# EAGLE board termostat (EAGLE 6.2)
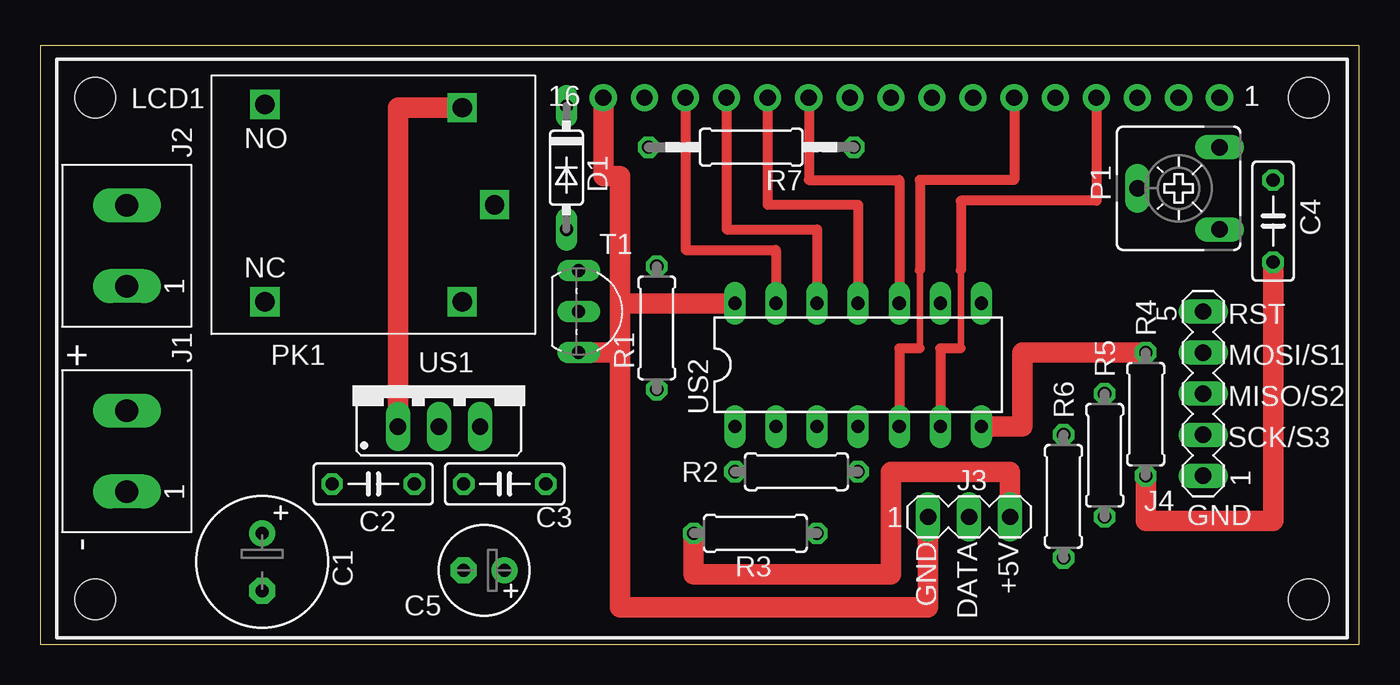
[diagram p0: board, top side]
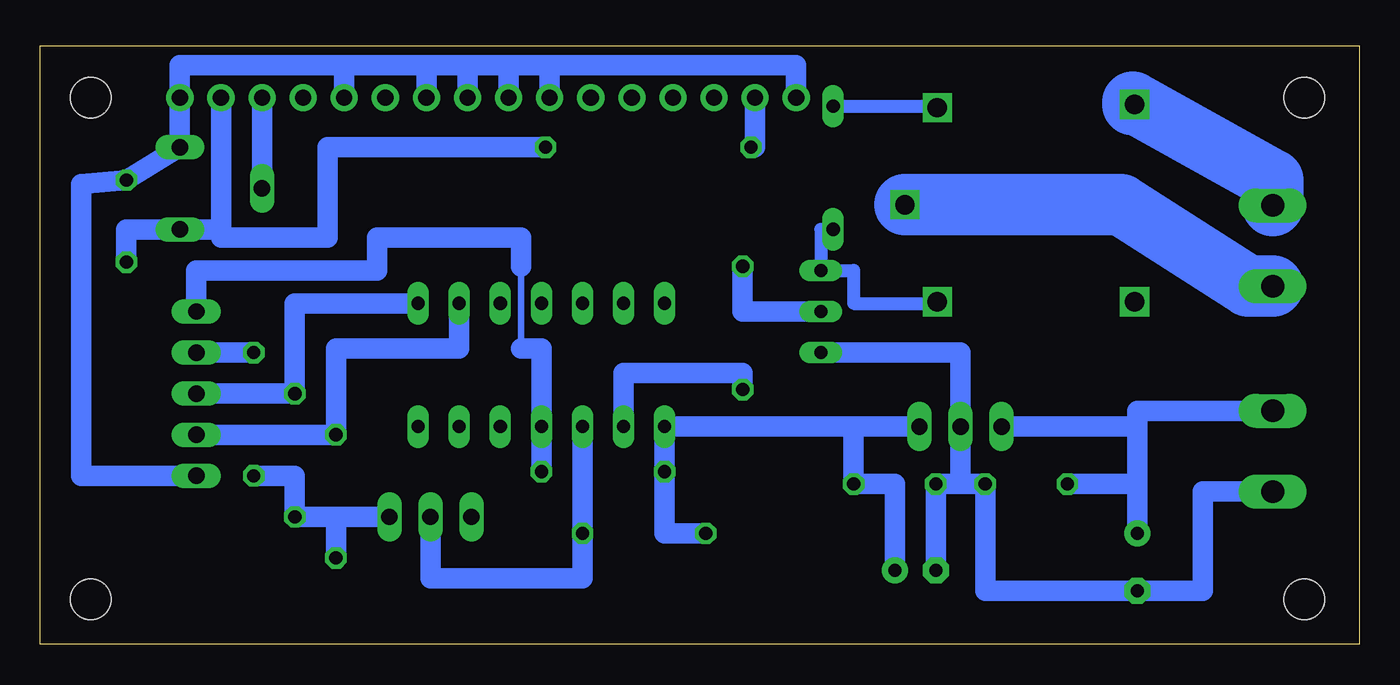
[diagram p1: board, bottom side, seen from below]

Size 81.51 x 37.01 mm. Coordinates in mm from the lower left corner, seen from the top.
Outline: 0,0 81.51,0 81.51,37.01 0,37.01 0,0
Copper layers (1*16): Top 0.035mm / dielectric 1.5mm / Bottom 0.035mm
Design rules: minimum track width 10mil, minimum drill 24mil, track to track 8mil, track to pad 8mil, pad to pad 8mil, via to via 8mil, smd to smd 8mil, copper to edge 40mil, drill to drill 8mil, minimum pad ring 10mil, minimum via ring 8mil, stop-mask expansion 4mil, vias tented up to drill 0mil, thermal gap 10mil

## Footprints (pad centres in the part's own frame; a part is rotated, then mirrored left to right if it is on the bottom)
E3,5-8 = drill 0.813 pad 1.6: + -1.778,0 | drill 0.813 pad 1.6 octagon: - 1.778,0
C050-025X075 = drill 0.813 octagon: 1 -2.54,0; 2 2.54,0
E2,5-6 = drill 0.813 pad 1.6: + -1.27,0 | drill 0.813 pad 1.6 octagon: - 1.27,0
DO35-7 = drill 0.813 long: A 3.81,0; C -3.81,0
2PIN-5MM = drill 1.4 long: P$1 -2.5,0; P$2 2.5,0
MA03-1 = drill 1.016 long: 1 -2.54,0; 2 0,0; 3 2.54,0
MA05-1 = drill 1.016 long: 1 -5.08,0; 2 -2.54,0; 3 0,0; 4 2.54,0; 5 5.08,0
LCD_HD44780_2X16_POD-SCIEZKAMI = drill 1 pad 1.676: 1 32,15.5; 2 29.46,15.5; 3 26.92,15.5; 4 24.38,15.5; 5 21.84,15.5; 6 19.3,15.5; 7 16.76,15.5; 8 14.22,15.5; 9 11.68,15.5; 10 9.14,15.5; 11 6.6,15.5; 12 4.06,15.5; 13 1.52,15.5; 14 -1.02,15.5; 15 -3.56,15.5; 16 -6.1,15.5 | hole 2.5: -37.5,-15.5; 37.5,-15.5; -37.5,15.5; 37.5,15.5
CA6V = drill 1.016 long: A -2.54,-2.54; E 2.54,-2.54; S 0,2.54
PK_POJED_JQC-3FG = drill 1.2 square: 1 5.5,6; 2 5.5,-6; C 7.5,0; NC -6.7,-6; NO -6.7,6.2
0207/7 = drill 0.813 octagon: 1 -3.81,0; 2 3.81,0
0207/12 = drill 0.813 octagon: 1 -6.35,0; 2 6.35,0
TO92-EBC = drill 0.813 long: B 0,-1.27; C -2.54,-1.27; E 2.54,-1.27
78XXS = drill 1.016 long: GND 0,-2.54; IN -2.54,-2.54; OUT 2.54,-2.54
DIL14 = drill 0.813 long: 1 -7.62,-3.81; 2 -5.08,-3.81; 3 -2.54,-3.81; 4 0,-3.81; 5 2.54,-3.81; 6 5.08,-3.81; 7 7.62,-3.81; 8 7.62,3.81; 9 5.08,3.81; 10 2.54,3.81; 11 0,3.81; 12 -2.54,3.81; 13 -5.08,3.81; 14 -7.62,3.81

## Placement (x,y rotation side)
C1  220u/35V  [E3,5-8]  13.72,5.08 270 top
C2  100n  [C050-025X075]  20.57,9.91 0 top
C3  100n  [C050-025X075]  28.7,9.91 180 top
C4  100n  [C050-025X075]  76.2,26.16 90 top
C5  100u/16V  [E2,5-6]  27.43,4.57 180 top
D1  1N4148  [DO35-7]  32.51,29.46 270 top
J1  ARK2-5MM  [2PIN-5MM]  5.33,11.94 90 top
J2  ARK2-5MM  [2PIN-5MM]  5.33,24.64 90 top
J3  [MA03-1]  57.4,7.87 0 top
J4  [MA05-1]  71.88,15.49 90 top
LCD1  1x16  [LCD_HD44780_2X16_POD-SCIEZKAMI]  40.89,18.29 0 top
P1  10k  [CA6V]  70.36,28.19 90 top
PK1  JQC-3FG  [PK_POJED_JQC-3FG]  20.57,27.18 0 top
R1  3,3k  [0207/7]  38.1,19.56 90 top
R2  3,3k  [0207/7]  46.74,10.67 180 top
R3  3,3k  [0207/7]  44.2,6.86 180 top
R4  3,3k  [0207/7]  68.33,14.22 90 top
R5  3,3k  [0207/7]  65.79,11.68 90 top
R6  3,3k  [0207/7]  63.25,9.14 90 top
R7  47  [0207/12]  43.94,30.73 180 top
T1  BC546  [TO92-EBC]  34.54,20.57 270 top
US1  7805  [78XXS]  24.64,16 0 top
US2  ATTINY24/44/84-PU  [DIL14]  50.55,17.27 0 top

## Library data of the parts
C1-C5 R1-R7 = rcl
D1 = diode
J1 J2 = zlacza_futrzak
J3 J4 = con-lstb; OC_FARNELL: unknown; OC_NEWARK: unknown
LCD1 PK1 = inne_futrzak
P1 = pot
T1 = transistor-npn
US1 = v-reg
US2 = scalaki_futrzak

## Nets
+5V: C3.1 C4.1 C5.+ J3.3 LCD1.2 P1.A R2.2 R3.2 R4.1 R5.1 R6.1 R7.1 US1.OUT US2.1
GND: C1.- C2.2 C3.2 C4.2 C5.- J1.P$1 J3.1 J4.1 LCD1.1 LCD1.5 LCD1.7 LCD1.8 LCD1.9 LCD1.10 LCD1.16 P1.E T1.E US1.GND US2.14
N$1: J4.5 R2.1 US2.4
N$31: C1.+ C2.1 D1.C J1.P$2 PK1.1 US1.IN
N$33: J2.P$2 PK1.NO
N$34: J2.P$1 PK1.C
N$35: J4.2 R6.2 US2.9
N$36: D1.A PK1.2 T1.C
N$38: J4.3 R5.2 US2.8
N$39: J3.2 R3.1 US2.3
N$40: J4.4 R4.2 US2.7
N$48: LCD1.3 P1.S
N$49: LCD1.15 R7.2
N$50: LCD1.14 US2.13
N$51: LCD1.13 US2.12
N$52: LCD1.4 US2.6
N$53: LCD1.6 US2.5
N$54: LCD1.12 US2.11
N$55: LCD1.11 US2.10
N$56: R1.2 T1.B
N$57: R1.1 US2.2

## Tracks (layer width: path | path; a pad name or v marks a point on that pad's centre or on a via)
+5V
  Top 1.27: R4.1 68.33,7.62 76.2,7.62 C4.1 | J3.3 59.94,10.67 52.58,10.67 52.58,4.32 40.39,4.32 R3.2
  Bottom 1.27: US1.OUT 31.24,13.46 | 31.24,13.46 C3.1 28.7,9.91 C5.+ | 31.24,13.46 US2.1 R2.2 42.93,6.86 R3.2 | 70.35,25.65 P1.A 76.2,25.65 C4.1 | 70.35,25.65 LCD1.2 | R4.1 65.79,10.41 R5.1 63.25,7.87 | R7.1 63.75,30.73 63.75,25.15 70.35,25.15 70.35,25.65 | J3.3 63.25,7.87 | 63.25,7.87 R6.1
GND
  Top 1.27: T1.E 35.81,18.03 | 35.81,18.03 35.81,21.08 | 35.81,21.08 35.81,28.96 34.79,28.96 LCD1.16 | US2.14 35.81,21.08 | J3.1 54.86,2.29 35.81,2.29 35.81,18.03
  Bottom 1.27: J1.P$1 9.65,9.44 9.65,3.3 C1.- 23.11,3.3 C2.2 24.64,9.91 | 24.64,9.91 C3.2 C5.- | 24.64,9.91 US1.GND 24.64,18.03 T1.E | 62.74,35.81 72.9,35.81 LCD1.1 72.89,30.99 P1.E C4.2 78.99,28.45 78.99,10.41 J4.1 | 62.74,35.81 62.73,35.81 | 62.73,35.81 LCD1.5 62.74,35.81 | 62.73,35.81 57.66,35.81 | 57.66,35.81 57.65,35.81 | 57.65,35.81 LCD1.7 57.66,35.81 | 57.65,35.81 55.12,35.81 | 55.12,35.81 55.11,35.81 | 55.11,35.81 LCD1.8 55.12,35.81 | 55.11,35.81 52.58,35.81 | 52.58,35.81 52.57,35.81 | 52.57,35.81 LCD1.9 52.58,35.81 | 52.57,35.81 50.04,35.81 | 50.04,35.81 50.03,35.81 | 50.03,35.81 LCD1.10 50.04,35.81 | 50.03,35.81 34.79,35.81 LCD1.16
N$1
  Bottom 0.406: 51.82,23.37 51.82,18.29
  Bottom 1.27: R2.1 US2.4 50.55,18.29 51.82,18.29 | J4.5 71.88,23.11 60.71,23.11 60.71,25.15 51.82,25.15 51.82,23.37
N$31
  Top 1.27: PK1.1 22.1,33.18 US1.IN
  Bottom 0.813: D1.C 26.07,33.27 PK1.1
  Bottom 1.27: J1.P$2 13.72,14.44 13.72,13.46 | 13.72,9.91 C1.+ | C2.1 13.72,9.91 | 13.72,9.91 13.72,13.46 | 13.72,13.46 US1.IN
N$33
  Bottom 3.81: PK1.NO 13.97,33.38 13.97,33.53 5.33,28.7 J2.P$2
N$34
  Bottom 3.81: J2.P$1 6.86,22.14 14.73,27.18 PK1.C
N$35
  Bottom 1.27: J4.2 R6.2 63.25,18.29 55.63,18.29 US2.9
N$36
  Bottom 0.813: D1.A 33.27,25.65 T1.C 31.24,23.11 31.24,21.08 26.16,21.08 26.16,21.34 26.07,21.34 PK1.2
N$38
  Bottom 1.27: J4.3 R5.2 65.79,21.08 US2.8
N$39
  Bottom 1.27: US2.3 R3.1 48.01,4.06 57.4,4.06 J3.2
N$40
  Top 1.27: R4.2 60.71,18.03 60.71,13.46 US2.7
  Bottom 1.27: J4.4 R4.2
N$48
  Bottom 1.27: P1.S 67.81,29.72 LCD1.3
N$49
  Bottom 1.27: R7.2 37.33,30.73 LCD1.15
N$50
  Top 0.61: LCD1.14 39.88,24.38 45.47,24.38 US2.13
N$51
  Top 0.61: LCD1.13 42.42,25.65 48.01,25.65 US2.12
N$52
  Top 0.406: 56.9,23.11 56.9,18.29
  Top 0.61: LCD1.4 65.28,27.43 56.9,27.43 56.9,23.11 | 56.9,18.29 55.63,18.29 US2.6
N$53
  Top 0.406: 54.36,23.11 54.36,18.29
  Top 0.61: LCD1.6 60.2,28.7 54.36,28.7 54.36,23.11 | 54.36,18.29 53.09,18.29 US2.5
N$54
  Top 0.61: LCD1.12 44.96,27.18 50.55,27.18 US2.11
N$55
  Top 0.61: LCD1.11 47.5,28.7 53.09,28.7 US2.10
N$56
  Bottom 1.27: T1.B 38.1,20.57 R1.2
N$57
  Bottom 1.27: R1.1 38.1,16.76 45.47,16.76 US2.2

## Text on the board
tPlace: RST | + | MOSI/S1 | MISO/S2 | SCK/S3 | - | GND | GND | DATA | +5V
